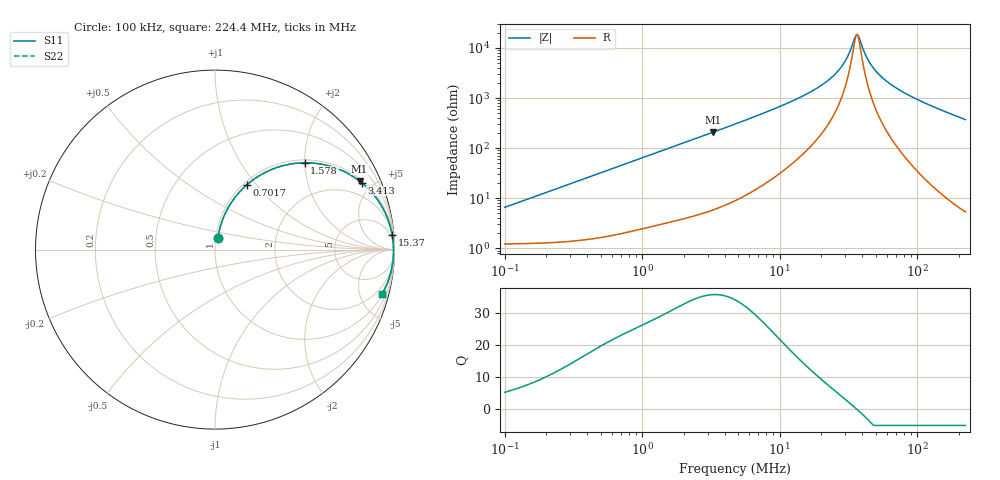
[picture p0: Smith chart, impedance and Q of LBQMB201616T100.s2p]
! LBQMB201616T100  S-PARAMETER MODEL  ( General Type )
! Model Generated by TAIYO YUDEN Corporation (http://www.ty-top.com)
! Version 1.0
! TAIYO YUDEN Control No. 191025NI43SB-FBB
! Copyright(c) 2019 TAIYO YUDEN CO.,LTD. All Rights Reserved.
! Product Description (link to TY-COMPAS)
! https://ds.yuden.co.jp/TYCOMPAS/or/detail?pn=LBQMB201616T100J&u=M
! Products Name : Inductors
! Characteristics :
!  Inductance : 10 uH , SRF(min) : 27 MHz , DC Resistance(max) : 1.56 Ohm , Rated Current : 215 mA
!  Case Size : 2.0 x 1.6 / 0.079 x 0.063 [mm/inch] , Thickness : 1.6 / 0.063 [mm/inch]
!  (Conditions: Temperature = 25 degC , DC Bias Current/Voltage = 0A / 0V)
! External Node Assignments :
!  1  o---GGG---o  2
! GND o---------o GND
! Frequency Range : 0.1MHz  -  224.402193MHz  [ 402 STEP ]
# MHz S RI R 50
! Freq[MHz].  S11 Real  S11 Imag  S21 Real  S21 Imag  S12 Real  S12 Imag  S22 Real  S22 Imag
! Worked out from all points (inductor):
!   401 points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, 100 kHz to 224.4 MHz, reference 50 ohm
!   read as one part in series: L = 10.3 uH near 103.9 kHz
!   highest Q = 35.6 at 3.284 MHz (marker M1), where L = 10.1 uH
!   self-resonance near 35.91 MHz
!   S11 on the Smith chart (normalised r, x): 100 kHz: 1.02, +0.13; 701.7 kHz: 1.04, +0.90; 1.578 MHz: 1.07, +2.00; 3.413 MHz: 1.12, +4.32; 15.37 MHz: 3, +23; 224.4 MHz: 1.11, -7.41
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0.1  0.0161 0.0627  0.9839 -0.0627  0.9839 -0.0627  0.0161 0.0627
0.364164  0.0642 0.2162  0.9358 -0.2162  0.9358 -0.2162  0.0642 0.2162
0.701672  0.1786 0.3618  0.8214 -0.3618  0.8214 -0.3618  0.1786 0.3618
1.326154  0.4177 0.476  0.5823 -0.476  0.5823 -0.476  0.4177 0.476
1.577583  0.4998 0.4838  0.5002 -0.4838  0.5002 -0.4838  0.4998 0.4838
3.283521  0.8052 0.3822  0.1948 -0.3822  0.1948 -0.3822  0.8052 0.3822
3.412675  0.8168 0.3731  0.1832 -0.3731  0.1832 -0.3731  0.8168 0.3731
4.737111  0.8942 0.2933  0.1058 -0.2933  0.1058 -0.2933  0.8942 0.2933
15.36545  0.9867 0.084  0.0133 -0.084  0.0133 -0.084  0.9867 0.084
17.25085  0.9889 0.0708  0.0111 -0.0708  0.0111 -0.0708  0.9889 0.0708
22.16762  0.9921 0.045  0.00789 -0.045  0.00789 -0.045  0.9921 0.045
26.88405  0.9936 0.027  0.0064 -0.027  0.0064 -0.027  0.9936 0.027
30.18284  0.9942 0.0166  0.00583 -0.0166  0.00583 -0.0166  0.9942 0.0166
35.21929  0.9946 0.00311  0.00539 -0.00311  0.00539 -0.00311  0.9946 0.00311
36.6046  0.9947 -0.000259  0.00534 0.000259  0.00534 0.000259  0.9947 -0.000259
38.04441  0.9947 -0.00363  0.0053 0.00363  0.0053 0.00363  0.9947 -0.00363
42.71263  0.9947 -0.0138  0.00533 0.0138  0.00533 0.0138  0.9947 -0.0138
47.03749  0.9945 -0.0224  0.00551 0.0224  0.00551 0.0224  0.9945 -0.0224
53.83777  0.994 -0.0349  0.00604 0.0349  0.00604 0.0349  0.994 -0.0349
62.8214  0.9929 -0.0501  0.00709 0.0501  0.00709 0.0501  0.9929 -0.0501
103.7348  0.984 -0.1092  0.016 0.1092  0.016 0.1092  0.984 -0.1092
224.4022  0.9291 -0.2496  0.0709 0.2496  0.0709 0.2496  0.9291 -0.2496
